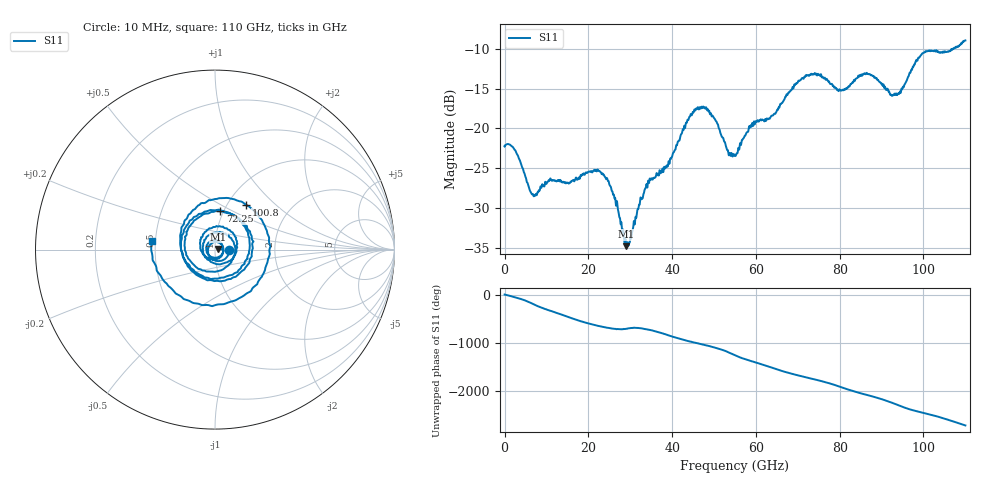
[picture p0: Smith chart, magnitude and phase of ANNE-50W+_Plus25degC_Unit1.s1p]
!Mini-Circuits Laboratory
!S-Parameters
!S1P File: Measurement
!Model: ANNE-50W+
!No.: Unit# 1 (U1_25°C)
!Run / Lot / Date Code: QN2409253 /  / 2409
!Fixture: N/A
!Network Analyzer: PNA-X N5242B;  Serial number: 74314
!Pin Outs: PORT<1> = pin<1>
!TEST CONDITIONS: Z:50 OHM SYSTEM, INPUT POWER = 0dBm, TEMP:25°C
!F-F adapter to 1FT F-M cable on Port 2 head. 1mm 1 PORT SmartCal
!Date: 9/5/2024 at 12:57:44 PM
# Hz  S  dB  R  50
!Frequency  S11 dB  S11 Deg
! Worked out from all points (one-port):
!   2208 points, 10 MHz to 110 GHz, reference 50 ohm
!   lowest |S11| = -34.8 dB at 29.05 GHz (marker M1), VSWR 1.04, Z = 51.8 + j0.437 ohm
!   |S11| at or under -10 dB: start of sweep to 107 GHz; 107.0983 GHz to 107.1912 GHz (92.94 MHz wide, 0.0867 % of centre)
!   S11 on the Smith chart (normalised r, x): 10 MHz: 1.17, +0.00; 72.25 GHz: 0.97, +0.43; 100.8 GHz: 1.22, +0.67; 110 GHz: 0.48, +0.05
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1e7  -22.26 0.1
6.8e9  -28.31 165.0
1.38e10  -26.81 -60.8
2.265e10  -25.37 66.2
2.755e10  -31.29 4.0
2.905e10  -34.82 13.4
3.415e10  -27.15 -5.7
4.13e10  -21.78 177.2
4.76e10  -17.41 40.0
5.18e10  -21.01 -60.0
5.505e10  -23.42 -176.6
5.83e10  -19.94 76.1
6.145e10  -18.93 -5.9
6.5e10  -17.75 -108.9
6.88e10  -14.79 156.8
7.225e10  -13.30 82.1
7.645e10  -13.62 -10.3
7.95e10  -15.12 -91.0
8.255e10  -14.47 179.3
8.61e10  -13.17 92.6
8.96e10  -14.19 6.9
9.305e10  -15.64 -97.4
9.63e10  -13.54 156.9
9.865e10  -11.27 99.0
1.0075e11  -10.32 55.2
1.035e11  -10.35 -7.1
1.063e11  -10.25 -82.7
1.1e11  -8.95 172.1
